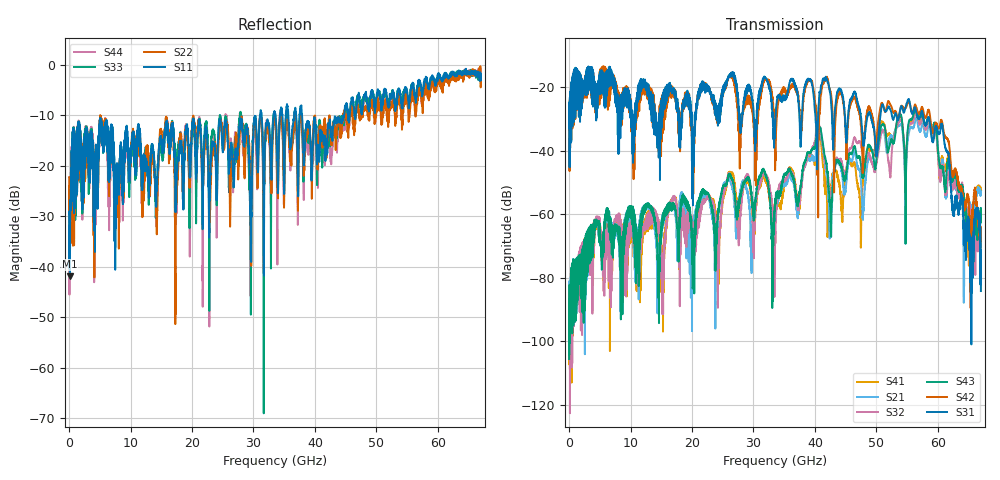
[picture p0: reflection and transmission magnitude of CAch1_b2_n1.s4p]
!Agilent Technologies,N5247A,US51170199,A.09.90.13
!Agilent N5247A: A.09.90.13
!Date: Wednesday, October 17, 2018 17:14:37
!Correction: S11(Full 4 Port(1,2,3,4))
!S12(Full 4 Port(1,2,3,4))
!S13(Full 4 Port(1,2,3,4))
!S14(Full 4 Port(1,2,3,4))
!S21(Full 4 Port(1,2,3,4))
!S22(Full 4 Port(1,2,3,4))
!S23(Full 4 Port(1,2,3,4))
!S24(Full 4 Port(1,2,3,4))
!S31(Full 4 Port(1,2,3,4))
!S32(Full 4 Port(1,2,3,4))
!S33(Full 4 Port(1,2,3,4))
!S34(Full 4 Port(1,2,3,4))
!S41(Full 4 Port(1,2,3,4))
!S42(Full 4 Port(1,2,3,4))
!S43(Full 4 Port(1,2,3,4))
!S44(Full 4 Port(1,2,3,4))
!S4P File: Measurements: <S11,S12,S13,S14>,
!<S21,S22,S23,S24>,
!<S31,S32,S33,S34>,
!<S41,S42,S43,S44>:
# Hz S  dB  R 50
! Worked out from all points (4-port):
!   6701 points, 10 MHz to 67 GHz, reference 50 ohm
!   strongest paths, dB at 10 MHz, 16.76 GHz, 33.51 GHz, 50.25 GHz, 67 GHz:
!     S31: -32.9, -22.0, -32.8, -37.5, -84.2
!     S42: -33.5, -21.1, -41.5, -31.6, -66.2
!     S43: -105.5, -58.5, -58.6, -39.4, -58.7
!     S32: -92.4, -56.5, -69.7, -41.5, -75.0
!     S21: -81.2, -58.3, -62.3, -38.2, -53.3
!     S41: -89.2, -56.2, -60.7, -37.2, -52.5
!   lowest |S11| = -41.9 dB at 140 MHz (marker M1), VSWR 1.02, Z = 50.1 - j0.799 ohm
!   |S11| at or under -10 dB: start of sweep to 31.04 GHz; 31.33 GHz to 33.31 GHz (1.979 GHz wide, 6.12 % of centre); 37.91 GHz to 44.63 GHz (6.72 GHz wide, 16.3 % of centre)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
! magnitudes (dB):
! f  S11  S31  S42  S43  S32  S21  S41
! 10 MHz  -29.4  -32.9  -33.5  -105.5  -92.4  -81.2  -89.2
! 140 MHz  -41.9  -24.5  -25.2  -100.5  -122.6  -96.2  -108.8
! 33.45 GHz  -9.2  -35.9  -38.9  -57.9  -73.8  -61.6  -59.7
! 40.73 GHz  -17.7  -21.6  -28.2  -32.7  -32.3  -33.9  -35.1
! 47.4 GHz  -7.6  -28.3  -30.0  -43.1  -37.5  -47.8  -60.1
! 56.43 GHz  -7.4  -27.3  -26.0  -27.0  -28.1  -29.8  -28.0
! 67 GHz  -3.0  -84.2  -66.2  -58.7  -75.0  -53.3  -52.5
